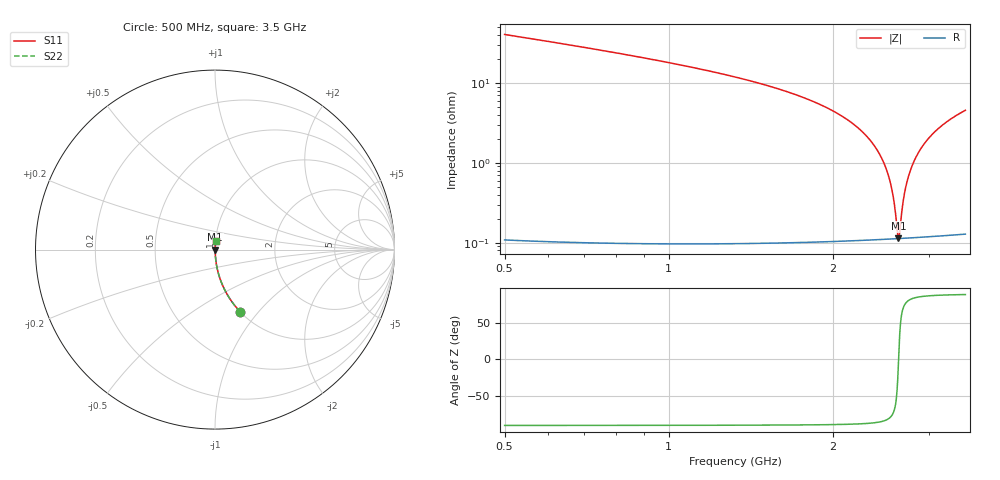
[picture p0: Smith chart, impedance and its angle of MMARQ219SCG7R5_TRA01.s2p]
! MMARQ219SCG7R5_TRA01  S-PARAMETER MODEL  ( General Type )
! Model Generated by TAIYO YUDEN Corporation (http://www.ty-top.com)
! Version 1.0
! TAIYO YUDEN Control No. 180601
! Copyright(c) 2018 TAIYO YUDEN CO.,LTD. All Rights Reserved.
! Product Description (link to TY-COMPAS)
! https://ds.yuden.co.jp/TYCOMPAS/or/detail?pn=MMARQ219SCG7R5CTRA01&u=M
! Products Name : Multilayer Ceramic Capacitors
! Characteristics :
!  Capacitance : 7.5 pF , Rated Voltage : 250V , TCC : CG / C0G
!  Case Size : 2.0 x 1.25 / 0.079 x 0.049 [mm/inch] , Thickness : 0.85 / 0.033 [mm/inch]
!  (Conditions: Temperature = 25 degC , DC Bias Current/Voltage = 0A / 0V)
! External Node Assignments :
!  1  o---| |---o  2
! GND o---------o GND
! Frequency Range : 500MHz  -  3500MHz  [ 401 STEP ]
# MHz S RI R 50
! Freq[MHz].  S11 Real  S11 Imag  S21 Real  S21 Imag  S12 Real  S12 Imag  S22 Real  S22 Imag
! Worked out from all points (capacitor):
!   401 points, 500 MHz to 3.5 GHz, reference 50 ohm
!   read as one part in series: C = 7.57 pF near 515 MHz
!   lowest |Z| = 113 mohm at 2.638 GHz (marker M1)
!   series resonance near 2.639 GHz, so ESL is about 480 pH
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500  0.1418 -0.3475  0.8582 0.3475  0.8582 0.3475  0.1418 -0.3475
710  0.0709 -0.2549  0.9291 0.2549  0.9291 0.2549  0.0709 -0.2549
1002.5  0.0321 -0.1735  0.9679 0.1735  0.9679 0.1735  0.0321 -0.1735
1505  0.00976 -0.0932  0.9902 0.0932  0.9902 0.0932  0.00976 -0.0932
2000  0.00302 -0.0446  0.997 0.0446  0.997 0.0446  0.00302 -0.0446
2172.5  0.00202 -0.0311  0.998 0.0311  0.998 0.0311  0.00202 -0.0311
2315  0.00151 -0.0209  0.9985 0.0209  0.9985 0.0209  0.00151 -0.0209
2420  0.00128 -0.0138  0.9987 0.0138  0.9987 0.0138  0.00128 -0.0138
2502.5  0.00117 -0.00847  0.9988 0.00847  0.9988 0.00847  0.00117 -0.00847
2540  0.00114 -0.0061  0.9989 0.0061  0.9989 0.0061  0.00114 -0.0061
2570  0.00113 -0.00424  0.9989 0.00424  0.9989 0.00424  0.00113 -0.00424
2592.5  0.00112 -0.00285  0.9989 0.00285  0.9989 0.00285  0.00112 -0.00285
2622.5  0.00112 -0.00102  0.9989 0.00102  0.9989 0.00102  0.00112 -0.00102
2637.5  0.00112 -0.000117  0.9989 0.000117  0.9989 0.000117  0.00112 -0.000117
2652.5  0.00113 0.000783  0.9989 -0.000783  0.9989 -0.000783  0.00113 0.000783
2682.5  0.00114 0.00257  0.9989 -0.00257  0.9989 -0.00257  0.00114 0.00257
2705  0.00115 0.0039  0.9989 -0.0039  0.9989 -0.0039  0.00115 0.0039
2765  0.0012 0.00738  0.9988 -0.00738  0.9988 -0.00738  0.0012 0.00738
2862.5  0.00133 0.0129  0.9987 -0.0129  0.9987 -0.0129  0.00133 0.0129
3005  0.00161 0.0206  0.9984 -0.0206  0.9984 -0.0206  0.00161 0.0206
3222.5  0.00224 0.0319  0.9978 -0.0319  0.9978 -0.0319  0.00224 0.0319
3500  0.00333 0.0453  0.9967 -0.0453  0.9967 -0.0453  0.00333 0.0453
